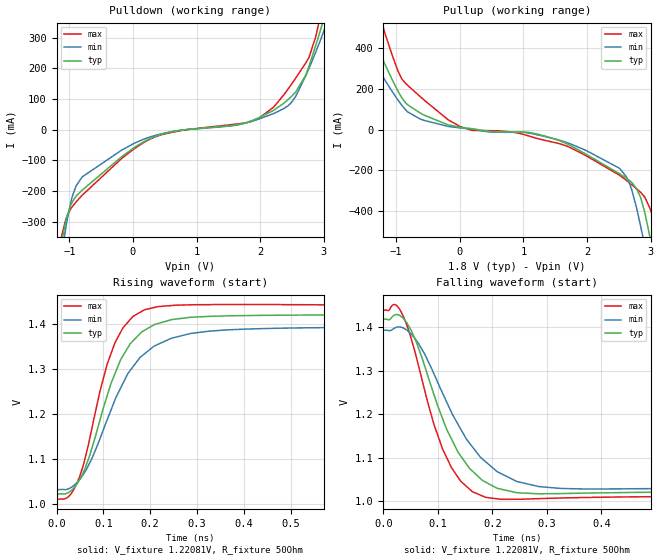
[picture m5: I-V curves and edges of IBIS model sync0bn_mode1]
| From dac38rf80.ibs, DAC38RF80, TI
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|   sync0bn_mode1 Model
[Model]   sync0bn_mode1
Model_type   Output
Polarity   Non-Inverting
Vmeas = 1.220813
Vref = 1.220813
Cref = 2pF
Rref = 200
|   typ   min   max
|   (nom PVT)   (fast PVT)   (slow PVT)
C_comp   6.491e-13   6.388e-13   7.043e-13
| Where nom  PVT is Nominal Process, 1.8V, 27C
|   Fast PVT is Strong Process,  1.89V, -40C
|   Slow PVT is Weak Process,   1.71V, 105C
[Voltage Range]   1.8   1.71   1.89
|Junction Temperature
[Temperature Range]   27   105   -40
[Pullup Reference]   1.8   1.71   1.89
[Pulldown Reference]   0   0   0
[Power Clamp Reference]   1.8   1.71   1.89
[GND Clamp Reference]   0   0   0
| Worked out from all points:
|   slope of the pulldown table from 0 to 0.27 V, typ, clamps not added: 8.4 ohm
|   slope of the pullup table from 0 to 0.27 V, typ, clamps not added: 23.2 ohm
|   falling waveform, V_fixture 1.22081V, R_fixture 50Ohm: 20-80 % time 75ps typ, 93.9ps min, 61.8ps max; typ from 1.42 V to 1.02 V
|   rising waveform, V_fixture 1.22081V, R_fixture 50Ohm: 20-80 % time 79.5ps typ, 98.4ps min, 63.7ps max; typ from 1.02 V to 1.42 V
[Pulldown]
|   Voltage   I(typ)   I(min)   I(max)
-1.8V     -1.511A    -1.418A    -1.667A
-1.119V   -368.8mA   -406.9mA   -344.9mA
-1.055V   -296.7mA   -320mA     -293.4mA
-972mV    -243.6mA   -232.7mA   -255.9mA
-796.2mV  -196.6mA   -153.5mA   -213mA
36.54mV   -56.08mA   -42.81mA   -59.74mA
493.2mV   -12.73mA   -11.26mA   -14.12mA
1.874V    30.04mA    27.69mA    27.85mA
2.381V    87.64mA    69.83mA    115.9mA
2.718V    178mA      175.8mA    217.8mA
2.985V    350.2mA    312.6mA    409.1mA
3.6V      896.3mA    1.265A     1.263A
[Pullup]
|   Voltage   I(typ)   I(min)   I(max)
-1.8V     837.3mA    987.6mA    1.296A
-1.598V   620.1mA    532.6mA    1.009A
-1.431V   498.3mA    378.7mA    773.4mA
-1.171V   317.8mA    240.5mA    468.6mA
-817.2mV  121.9mA    87.31mA    217.4mA
36mV      11.25mA    8.13mA     11.94mA
1.976V    -118.7mA   -100.4mA   -126mA
2.62V     -237.9mA   -231.4mA   -248.5mA
2.91V     -407.5mA   -571.7mA   -331.7mA
2.99V     -528.1mA   -689.7mA   -386mA
3.146V    -794.9mA   -922.2mA   -617mA
3.6V      -1.568A    -1.6A      -1.544A
[Ramp]
R_load = 50
|   typ   min   max
dV/dt_r   0.100884/1.62599e-10  0.0988105/1.69933e-10   0.557957/1.40127e-10
dV/dt_f   0.237329/7.49999e-11   0.216367/9.37077e-11   0.256973/6.18437e-11
[Falling Waveform]
V_fixture = 1.22081V
V_fixture_min = 1.21309V
V_fixture_max = 1.22558V
R_fixture = 50Ohm
|   Time   V(typ)   V(min)   V(max)
0s        1.419V     1.393V     1.44V
22.11ps   1.429V     1.4V       1.452V
42.66ps   1.411V     1.394V     1.406V
75.82ps   1.311V     1.338V     1.255V
108.5ps   1.19V      1.249V     1.121V
141.5ps   1.105V     1.167V     1.047V
187.9ps   1.044V     1.091V     1.009V
245.2ps   1.02V      1.046V     1.005V
325.2ps   1.018V     1.03V      1.008V
1.045ns   1.023V     1.032V     1.012V
[Rising Waveform]
V_fixture = 1.22081V
V_fixture_min = 1.21309V
V_fixture_max = 1.22558V
R_fixture = 50Ohm
|   Time   V(typ)   V(min)   V(max)
0s        1.023V     1.033V     1.012V
25.38ps   1.026V     1.035V     1.017V
49.45ps   1.055V     1.055V     1.062V
92.78ps   1.187V     1.146V     1.251V
124.9ps   1.29V      1.232V     1.358V
157.6ps   1.356V     1.297V     1.41V
187.9ps   1.386V     1.334V     1.431V
245.2ps   1.409V     1.368V     1.441V
365.2ps   1.418V     1.387V     1.443V
1.014ns   1.419V     1.394V     1.44V
